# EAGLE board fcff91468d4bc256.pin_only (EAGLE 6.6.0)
REV: B

Size 40.64 x 44.45 mm. Coordinates in mm from the lower left corner, seen from the top.
Outline: 0,0 40.64,0 40.64,41.91 arc90 38.1,44.45 2.54,44.45 arc90 0,41.91 0,11.18 1.27,11.18 1.27,7.62 0,7.62 0,0
Copper layers (1*16): Top 0.035mm / dielectric 1.5mm / Bottom 0.035mm
Design rules "adafruit *": minimum track width 8mil, minimum drill 15.5mil, track to track 8mil, track to pad 8mil, pad to pad 8mil, via to via 8mil, smd to smd 8mil, copper to edge 10mil, drill to drill 8mil, minimum pad ring 10mil, minimum via ring 8mil, stop-mask expansion 2mil, vias tented up to drill 20mil, thermal gap 10mil

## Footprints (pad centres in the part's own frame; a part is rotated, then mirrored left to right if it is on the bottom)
1X01-CLEANBIG = drill 1.016 pad 1.778: 1 0,0
0805-NO = smd 1.3 x 1.5: 1 -0.95,0; 2 0.95,0
C1210 = smd 1.6 x 2.7: 1 -1.4,0; 2 1.4,0
RESPACK_4X0603 = smd 0.45 x 0.9: 1 -1.3,-0.85; 2 -0.4,-0.85; 3 0.4,-0.85; 4 1.3,-0.85; 5 1.3,0.85; 6 0.4,0.85; 7 -0.4,0.85; 8 -1.3,0.85
CHIPLED_0805_NOOUTLINE = smd 1.2 x 1.2: A 0,-1.05; C 0,1.05
JSTPH2 = smd 1 x 4.6: 1 -1,-3.7; 2 1,-3.7 | smd 1.6 x 3.4: NC1 -3.4,1.5; NC2 3.4,1.5
SOD-123 = smd 1.4 x 1.4: A 1.85,0; C -1.85,0
SOT363 = smd 0.5 x 0.5: 1 -0.75,-0.9; 3 0.75,-0.9; 4 0.75,0.9; 6 -0.75,0.9 | smd 0.4 x 0.5: 2 0,-0.9; 5 0,0.9
SOD-323 = smd 1.35 x 0.8: A 1.27,0; C -1.27,0
FIDUCIAL_1MM = smd 1 x 1: 1 0,0
TSSOP14 = smd 0.35 x 0.9: 1 -1.95,-2.925; 2 -1.3,-2.925; 3 -0.65,-2.925; 4 0,-2.925; 5 0.65,-2.925; 6 1.3,-2.925; 7 1.95,-2.925; 8 1.95,2.925; 9 1.3,2.925; 10 0.65,2.925; 11 0,2.925; 12 -0.65,2.925; 13 -1.3,2.925; 14 -1.95,2.925
1X02_ROUND = drill 1 pad 1.778: 1 -1.27,0; 2 1.27,0
1X16_ROUND = drill 1 pad 1.676: 1 -19.05,0; 2 -16.51,0; 3 -13.97,0; 4 -11.43,0; 5 -8.89,0; 6 -6.35,0; 7 -3.81,0; 8 -1.27,0; 9 1.27,0; 10 3.81,0; 11 6.35,0; 12 8.89,0; 13 11.43,0; 14 13.97,0; 15 16.51,0; 16 19.05,0
SC59-BEC = smd 1 x 1.4: B -0.95,-1.2; C 0,1.2; E 0.95,-1.2
BTN_KMR2_4.6X2.8 = smd 0.9 x 1: A 2.05,0.8; A' -2.05,0.8; B 2.05,-0.8; B' -2.05,-0.8
TP11R = smd 1.1 x 1.1: TP 0,0
SOT23-5 = smd 0.55 x 1.2: 1 -0.95,-1.3; 2 0,-1.3; 3 0.95,-1.3; 4 0.95,1.3; 5 -0.95,1.3
SIM900_SMT = smd 2 x 0.6: P$1 -12.4,8; P$2 -12.4,7; P$3 -12.4,6; P$4 -12.4,5; P$5 -12.4,4; P$6 -12.4,3; P$7 -12.4,2; P$8 -12.4,1; P$9 -12.4,0; P$10 -12.4,-1; P$11 -12.4,-2; P$12 -12.4,-3; P$13 -12.4,-4; P$14 -12.4,-5; P$15 -12.4,-6; P$16 -12.4,-7; P$17 -12.4,-8; P$35 12.4,-8; P$36 12.4,-7; P$37 12.4,-6; P$38 12.4,-5; P$39 12.4,-4; P$40 12.4,-3; P$41 12.4,-2; P$42 12.4,-1; P$43 12.4,0; P$44 12.4,1; P$45 12.4,2; P$46 12.4,3; P$47 12.4,4; P$48 12.4,5; P$49 12.4,6; P$50 12.4,7; P$51 12.4,8 | smd 0.6 x 2: P$18 -8,-12.4; P$19 -7,-12.4; P$20 -6,-12.4; P$21 -5,-12.4; P$22 -4,-12.4; P$23 -3,-12.4; P$24 -2,-12.4; P$25 -1,-12.4; P$26 0,-12.4; P$27 1,-12.4; P$28 2,-12.4; P$29 3,-12.4; P$30 4,-12.4; P$31 5,-12.4; P$32 6,-12.4; P$33 7,-12.4; P$34 8,-12.4; P$52 8,12.4; P$53 7,12.4; P$54 6,12.4; P$55 5,12.4; P$56 4,12.4; P$57 3,12.4; P$58 2,12.4; P$59 1,12.4; P$60 0,12.4; P$61 -1,12.4; P$62 -2,12.4; P$63 -3,12.4; P$64 -4,12.4; P$65 -5,12.4; P$66 -6,12.4; P$67 -7,12.4; P$68 -8,12.4
MOUNTINGHOLE_2.5_PLATED = drill 2.5 pad 3.2: P$1 0,0
SMA_EDGELAUNCH_UFL = smd 4.064 x 1.524: GND@1 2.032,-2.54; GND@2 2.032,2.54 | smd 4.064 x 1.524 bottom: GND@3 2.032,2.54; GND@4 2.032,-2.54 | smd 2.032 x 1.016: P 3.048,0
4UCONN_20329 = smd 1 x 2: BASE@1 -0.75,-2; BASE@2 0.75,-2 | smd 0.4 x 1.35: D+ 0,0.775; D- -0.65,0.775; GND 1.3,0.775; ID 0.65,0.775; VBUS -1.3,0.775 | drill 0.7 offset: SPRT@1 -3.3,0.9; SPRT@2 3.3,0.9 | drill 0.6 pad 2.5 square: SPRT@3 -3.6,-1.9; SPRT@4 3.6,-1.9 | hole 0.7: -1.95,0; 1.95,0
U.FL = smd 2.2 x 1.05: 1 0,1.375; 2 0,-1.375 | smd 0.8 x 1: 3 1.525,0
4UCONN_18510 = smd 1.5 x 2.5: 1-GND 2.8,-3.3; 2-TIP 9.3,3.4; 3-OUTER_SLEEVE 5.5,-3.3 | smd 1.5 x 3.4: 4-INNER_SLEEVE 2.8,2.9 | hole 1.3: 10.5,0
C707_10M006_512_2 = smd 1.7 x 1.3: C1 -12.85,-3.915; C2 -12.85,-1.375; C3 -12.85,1.165; C5 12.85,-3.915; C6 12.85,-1.375; C7 12.85,1.165

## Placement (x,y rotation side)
ADC1  [1X01-CLEANBIG]  32.51,9.91 0 top
C1  10µF  [0805-NO]  8.13,19.05 0 top
C5  10pF  [0805-NO]  11.54,39.51 0 top
C6  33pF  [0805-NO]  10.88,37.42 0 top
C7  100uF  [C1210]  10.54,29.46 270 top
C9  10uF  [0805-NO]  8.13,16.76 180 top
C11  10uF  [0805-NO]  11.43,14.73 90 top
C14  33pF  [RESPACK_4X0603]  31.88,6.35 270 top
C15  10pF  [RESPACK_4X0603]  28.7,6.35 270 top
C16  33pF  [RESPACK_4X0603]  35.31,6.35 90 top
C17  10pF  [RESPACK_4X0603]  38.48,6.35 90 top
CHRG  ORANGE  [CHIPLED_0805_NOOUTLINE]  2.41,26.81 270 top
CN2  JSTPH  [JSTPH2]  3.81,34.16 90 top
D1  MMSZ5231BT1G  [SOD-123]  6.73,39.62 180 top
D2  SMF05C  [SOT363]  29.21,10.03 270 top
D3  1N4148  [SOD-323]  34.92,41.78 270 top
D4  1N4148  [SOD-323]  14.48,7.24 90 top
D5  1N4148  [SOD-323]  17.14,7.37 90 top
D6  1N4148  [SOD-323]  13.34,10.67 90 top
D7  1N4148  [SOD-323]  15.88,10.67 90 top
DONE  GREEN  [CHIPLED_0805_NOOUTLINE]  2.42,28.66 90 top
FID1  FIDUCIAL""  [FIDUCIAL_1MM]  35.69,35.18 0 top
FID2  FIDUCIAL""  [FIDUCIAL_1MM]  2.29,34.92 0 top
FID3  FIDUCIAL""  [FIDUCIAL_1MM]  5.59,9.53 0 top
FID4  FIDUCIAL""  [FIDUCIAL_1MM]  1.78,37.59 0 bottom
FID5  FIDUCIAL""  [FIDUCIAL_1MM]  34.04,24.13 0 bottom
IC1  74VHCT125PW  [TSSOP14]  22.23,8.38 90 top
JP3  BUZZ  [1X02_ROUND]  33.15,41.91 90 top
JP10  [1X16_ROUND]  20.32,1.65 0 top
NETSTAT  RED  [CHIPLED_0805_NOOUTLINE]  26.04,42.55 270 top
PWM  [1X01-CLEANBIG]  39.12,35.43 0 top
PWRSTAT  BLUE  [CHIPLED_0805_NOOUTLINE]  30.1,42.55 270 top
Q1  DTC143ZUAT106  [SC59-BEC]  38.1,38.23 90 top
R1  470  [0805-NO]  5.97,26.92 0 top
R2  1K  [0805-NO]  5.99,28.7 0 top
R3  2K  [0805-NO]  11.05,19.81 270 top
R4  1K  [0805-NO]  30.1,40.89 0 top
R5  1K  [0805-NO]  26.16,40.89 0 top
R6  10K  [0805-NO]  10.79,23.37 90 top
SW1  KMR2  [BTN_KMR2_4.6X2.8]  10.79,42.55 0 top
TP1  TPTP11R  [TP11R]  10.79,25.78 0 top
U2  MCP73831T-2ACI/OT  [SOT23-5]  8.13,22.61 180 top
U3  SIM808  [SIM900_SMT]  25.78,25.27 0 top
U$21  [ADAFRUIT_2.5MM]  5.97,13.08 0 top
U$25  [PCBFEAT-REV-040]  7.87,40.89 0 bottom
U$26  [FONA_LOGO]  19.68,27.94 0 bottom
U$33  MOUNTINGHOLE2.5  [MOUNTINGHOLE_2.5_PLATED]  38.1,41.91 90 top
U$34  MOUNTINGHOLE2.5  [MOUNTINGHOLE_2.5_PLATED]  2.54,41.91 90 top
U$36  [ADAFRUIT_5MM]  14.86,38.99 0 bottom
X1  uFL  [SMA_EDGELAUNCH_UFL]  19.81,44.32 270 top
X2  MicroB  [4UCONN_20329]  4.32,20.07 270 top
X3  uFL  [U.FL]  38.35,10.92 90 top
X4  4UCONN_18510  [4UCONN_18510]  0.13,9.4 0 top
X6  SIM_LOCKAMPHENOL  [C707_10M006_512_2]  28.45,24.77 270 bottom

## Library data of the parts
ADC1 PWM = adafruit
C1 C5 C6 C9 C11 C14-C17 CHRG CN2 D1-D3 D7 DONE JP3 JP10 NETSTAT PWRSTAT R1-R6 SW1 U2 U3 U$21 U$25 U$26 U$36 X1-X4 = microbuilder
C7 = rcl
D4-D6 = microbuilder; COMPANY: ADAFRUIT INDUSTRIES; DRAWN: KTOWN; REV: A
FID1-FID5 U$33 U$34 = microbuilder; BOM: EXCLUDE
IC1 = 74xx-us
Q1 = transistor
TP1 = testpad
X6 = microbuilder; OC_FARNELL: unknown; OC_NEWARK: unknown

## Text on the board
tPlace: Key | Net | PWR | GSM ANT | PWM1 | 2.8V | GPS / ANT | ADC | Bat | GND | NS | Mic | 5V | Vio | Rst | RX | TX | RTS | Key | RI | PStat | + | - | + | SPKR | -
bPlace: Buzzer | + | - | FONA+GPS | GSM Cell-Phone | with GPS | adafruit! | Data/Voice/SMS | GPS uses 50ohm / Passive Ant. | 3.7V LiPoly | Req. during use | USB Charging | @500mA | CTIA Headset / TRRS: LR-M | 2G GSM / SIM Card | Vio: I/O Level 3-5VDC

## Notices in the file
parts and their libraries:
microbuilder: This work is placed in the public domain, and may be freely used for commercial and non-commercial work with the following conditions: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
